(* Logix 5000 Routine export ModbusRouter; software revision 19.01 *)

TYPE AparianModbusMessageResponse :
STRUCT
   Status : INT;
   ResponseLength : INT;
   Response : SINT[255];
END_STRUCT
END_TYPE

TYPE AparianModbusRouterInput :
STRUCT
   Instance : STRING;
   Status : AparianModbusRouterStatus;
   TransactionRate : DINT;
   Temperature : REAL;
   ModbusRxPacketCount : DINT;
   ModbusTxPacketCount : DINT;
   ModbusChecksumErrors : DINT;
   ModbusTimeout : DINT;
   ModbusUnspecifiedErrors : DINT;
   TagReads : DINT;
   TagWrites : DINT;
   TagConnectionFailures : DINT;
   TagErrors : DINT;
END_STRUCT
END_TYPE

TYPE AparianModbusMessageRequest :
STRUCT
   DestinationAddress : INT;
   Function : INT;
   Port : INT;
   RequestSize : INT;
   IPAddress : INT[4];
   RequestData : SINT[256];
END_STRUCT
END_TYPE

TYPE AparianModbusRouterOutput :
STRUCT
   RoutingInhibited : BOOL;
END_STRUCT
END_TYPE

TYPE AparianModbusRouterStatus :
STRUCT
   ReactiveTagMode : BOOL;
   ScheduledTagMode : BOOL;
   UnscheduledMode : BOOL;
   ConfigurationValid : BOOL;
   RoutingInhibited : BOOL;
   Reserved1 : BOOL;
   Reserved2 : BOOL;
   Reserved3 : BOOL;
   ScheduledTagStatus0 : BOOL;
   ScheduledTagStatus1 : BOOL;
   ScheduledTagStatus2 : BOOL;
   ScheduledTagStatus3 : BOOL;
   ScheduledTagStatus4 : BOOL;
   ScheduledTagStatus5 : BOOL;
   ScheduledTagStatus6 : BOOL;
   ScheduledTagStatus7 : BOOL;
   ScheduledTagStatus8 : BOOL;
   ScheduledTagStatus9 : BOOL;
   ScheduledTagStatus10 : BOOL;
   ScheduledTagStatus11 : BOOL;
   ScheduledTagStatus12 : BOOL;
   ScheduledTagStatus13 : BOOL;
   ScheduledTagStatus14 : BOOL;
   ScheduledTagStatus15 : BOOL;
   ScheduledTagStatus16 : BOOL;
   ScheduledTagStatus17 : BOOL;
   ScheduledTagStatus18 : BOOL;
   ScheduledTagStatus19 : BOOL;
END_STRUCT
END_TYPE

VAR_GLOBAL   (* controller tags *)
   ModbusMessageResponse : AparianModbusMessageResponse := (ResponseLength := 5, Response[0] := 4, Response[1] := 22, Response[2] := 46);
   SendModbusMSG : BOOL;
   MBR01Output : AparianModbusRouterOutput;
   ModbusMSG : MESSAGE;
        MessageParameters(MessageType := CIP Generic, RequestedLength := 272, ConnectedFlag := 2, ConnectionPath := MBR01, ServiceCode := 16#006a, ObjectType := 16#040e, TargetObject := 1, LocalElement := ModbusMessageRequest, DestinationTag := ModbusMessageResponse)
   ModbusMessageRequest : AparianModbusMessageRequest := (DestinationAddress := 1, Function := 3, Port := 1, RequestSize := 4, IPAddress[0] := 192, IPAddress[1] := 168, IPAddress[2] := 1, IPAddress[3] := 219, RequestData[3] := 2);
   MBR01Input : AparianModbusRouterInput := (Instance := 'ModbusSample', Temperature := 39.5513, ModbusRxPacketCount := 3, ModbusTxPacketCount := 5);
END_VAR

PROGRAM MainProgram

ROUTINE ModbusRouter   (* ladder *)
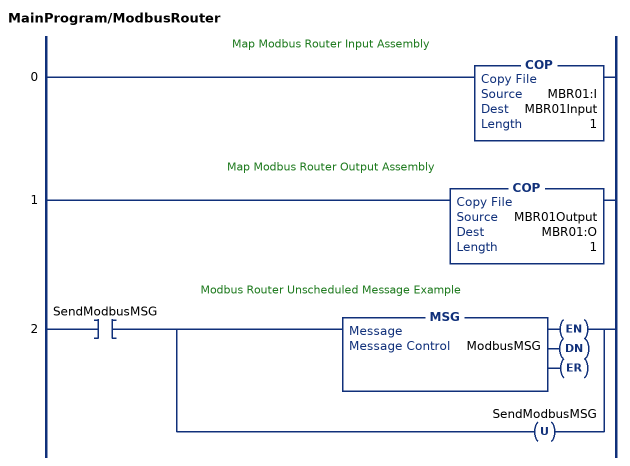
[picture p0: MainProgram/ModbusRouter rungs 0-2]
   // Map Modbus Router Input Assembly
   0: COP(MBR01:I,MBR01Input,1);
   // Map Modbus Router Output Assembly
   1: COP(MBR01Output,MBR01:O,1);
   // Modbus Router Unscheduled Message Example
   2: XIC(SendModbusMSG)[MSG(ModbusMSG) ,OTU(SendModbusMSG) ];
END_ROUTINE
END_PROGRAM
